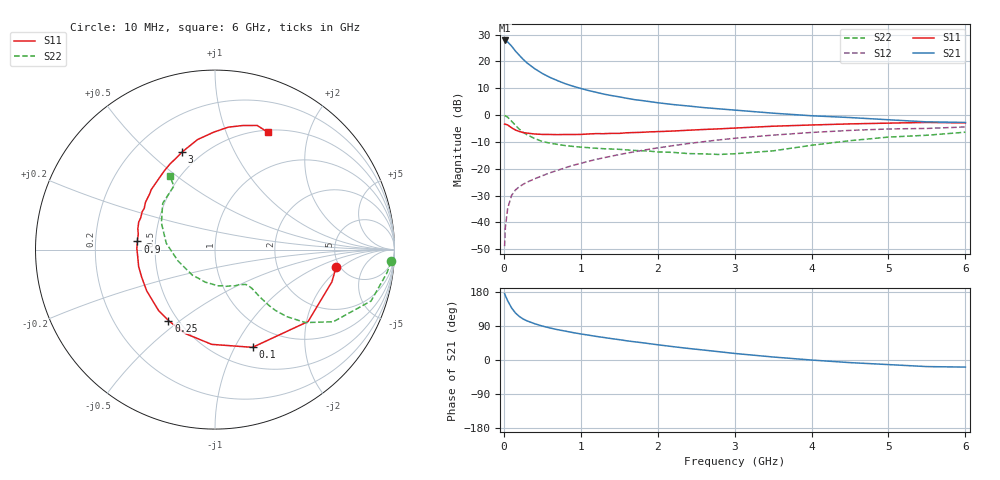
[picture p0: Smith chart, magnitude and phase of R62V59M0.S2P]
! SIEMENS Small Signal Semiconductors
! BFR193
! Si NPN RF Bipolar Junction Transistor in SOT23
! VCE = 2.5 V  IC = 9 mA
! Common Emitter S-Parameters:  May  1996
# GHz  S  MA  R  50
!  f  S11  S21  S12  S22
! GHz  MAG  ANG  MAG  ANG  MAG  ANG  MAG  ANG
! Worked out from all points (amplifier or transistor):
!   36 points, 10 MHz to 6 GHz, reference 50 ohm
!   highest |S21| = 27.8 dB at 10 MHz (marker M1)
!   |S21| within 3 dB of that: start of sweep to 125.2 MHz
!   unconditionally stable (mu >= 1): 728.4 MHz to 2.025 GHz
!   at 250 MHz: K = 0.62, MSG = 23.3 dB, |S12| = -25.8 dB
!   at 1.4 GHz: K = 1.04, MAG = 10.0 dB, |S12| = -15.3 dB
!   at 6 GHz: K = 0.96, MSG = 0.8 dB, |S12| = -4.4 dB
!   S11 on the Smith chart (normalised r, x): 10 MHz: 4.66, -1.67; 100 MHz: 0.72, -1.18; 250 MHz: 0.45, -0.45; 900 MHz: 0.39, +0.04; 3 GHz: 0.40, +0.64; 6 GHz: 0.53, +1.41
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0.01  0.6816 -8.1  24.67 175.1  0.0036 86.8  0.9829 -3.8
0.02  0.6758 -15.4  24.18 170.0  0.0081 83.3  0.9674 -7.6
0.05  0.6553 -37.7  23.09 156.2  0.0183 74.1  0.9156 -18.2
0.1  0.5833 -69.0  19.42 137.7  0.0317 63.4  0.7717 -31.4
0.15  0.5283 -92.0  15.73 124.3  0.0401 56.9  0.6474 -38.9
0.2  0.4959 -110.0  13.1 115.1  0.0462 54.8  0.5481 -43.0
0.25  0.4728 -123.3  11 108.3  0.0512 53.9  0.4775 -45.2
0.3  0.4624 -132.9  9.429 103.3  0.056 54.4  0.4317 -46.0
0.4  0.4446 -148.8  7.359 95.8  0.0649 55.6  0.3657 -46.5
0.5  0.4365 -159.3  5.978 89.6  0.0741 57.8  0.3222 -46.5
0.6  0.4358 -167.5  5.045 84.5  0.0841 59.4  0.2995 -46.4
0.7  0.4323 -175.0  4.38 80.0  0.0937 60.3  0.2846 -46.8
0.9  0.4349 174.0  3.456 72.3  0.1159 61.6  0.2608 -48.3
1.1  0.4454 164.8  2.876 65.6  0.1376 62.0  0.2473 -52.1
1.3  0.4506 156.8  2.464 59.4  0.1605 61.5  0.2362 -55.8
1.6  0.4684 145.8  2.058 50.6  0.1955 59.8  0.2245 -64.4
2.2  0.505 128.1  1.574 35.2  0.2697 54.3  0.2019 -86.2
3  0.5734 108.7  1.241 17.3  0.3696 43.6  0.1903 -131.4
3.5  0.6207 99.0  1.087 7.9  0.4238 36.0  0.2155 -163.0
4.5  0.6862 83.8  0.901 -6.9  0.519 20.7  0.3338 153.5
5.5  0.7305 71.2  0.748 -17.4  0.5644 5.1  0.4214 122.9
6  0.7168 65.7  0.73 -18.7  0.6015 0.5  0.48 121.6
